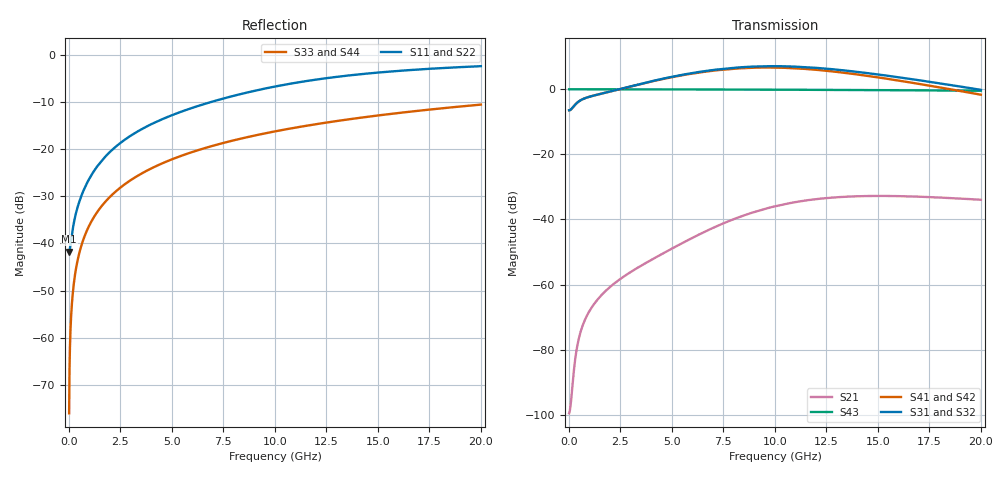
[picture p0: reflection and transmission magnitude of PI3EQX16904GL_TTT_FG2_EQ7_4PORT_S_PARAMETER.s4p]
! NPort=4 DATA=2000 NOISE=0 GROUPDELAY=0 COMPLEX_DATAFORMAT=POLAR
! NumOfBlock=1 NumOfParam=0
! .MODEL Smodel S TSTONEFILE=PI3EQX16904GL_TTT_FG2_EQ7_4PORT_S_PARAMETER.s4p TYPE=S
!  -- The above .MODEL line can be used for the S element in the netlist.
! The s parameter is extracted from the linear redriver, it is not bi-directional; only s(4,1)s(4,2) and s(3,1)s(3,2)
! should be the insertion loss
!Port definition:
!Port1 = input+
!Port2 = input-
!Port3 = output+
!Port4 = output-
# Hz S MA R  50
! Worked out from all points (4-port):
!   2000 points, 10 MHz to 20 GHz, reference 50 ohm
!   strongest paths, dB at 10 MHz, 5.01 GHz, 10.01 GHz, 15.01 GHz, 20 GHz:
!     S31: -6.5, 3.9, 7.1, 4.6, -0.2
!     S32: -6.5, 3.8, 7.1, 4.5, -0.2
!     S41: -6.5, 3.7, 6.7, 3.7, -1.7
!     S42: -6.5, 3.7, 6.6, 3.6, -1.7
!     S43: 0.0, 0.0, -0.1, -0.3, -0.4
!     S21: -99.6, -48.9, -35.9, -32.8, -33.9
!   lowest |S11| = -41.7 dB at 10 MHz (marker M1), VSWR 1.02, Z = 49.2 - j0.0603 ohm
!   |S11| at or under -10 dB: start of sweep to 6.858 GHz
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1e7  0.008182 -175.7  1.05e-05 7.8  0 0.0  0 0.0
     1.05e-05 7.8  0.008182 -175.7  0 0.0  0 0.0
     0.4744 0.7  0.4744 -179.3  0.0001571 -90.0  1 -0.0
     0.4744 -179.3  0.4744 0.7  1 -0.0  0.0001571 -90.0
2.8e8  0.01832 -124.6  6.153e-05 116.3  0 0.0  0 0.0
       6.153e-05 116.3  0.01832 -124.6  0 0.0  0 0.0
       0.5696 14.2  0.5696 -165.8  0.004398 -90.3  1 -0.3
       0.5695 -166.3  0.5696 13.7  1 -0.3  0.004398 -90.3
1.01e9  0.04965 -106.4  0.0003975 112.2  0 0.0  0 0.0
        0.0003974 112.2  0.04965 -106.4  0 0.0  0 0.0
        0.7708 11.7  0.7715 -168.3  0.01586 -90.9  0.9999 -0.9
        0.7704 -170.1  0.771 9.9  0.9999 -0.9  0.01586 -90.9
5.5e9  0.2531 -103.9  0.00436 110.5  0 0.0  0 0.0
       0.004328 110.9  0.2531 -103.9  0 0.0  0 0.0
       1.67 -30.1  1.658 149.5  0.08605 -95.1  0.996 -4.9
       1.644 140.1  1.633 -40.3  0.996 -4.9  0.08605 -95.1
9.41e9  0.4369 -111.2  0.01432 74.7  0 0.0  0 0.0
        0.01423 75.7  0.4368 -111.2  0 0.0  0 0.0
        2.258 -96.8  2.243 83.0  0.1461 -98.7  0.9884 -8.4
        2.162 66.8  2.148 -113.4  0.9884 -8.4  0.1461 -98.7
1.332e10  0.5999 -121.7  0.02231 23.1  0 0.0  0 0.0
          0.02224 24.5  0.6 -121.6  0 0.0  0 0.0
          1.958 -165.7  1.945 14.0  0.2044 -102.3  0.9772 -11.8
          1.801 -8.4  1.789 171.4  0.9772 -11.8  0.2044 -102.3
2e10  0.7643 -136.5  0.02007 -39.0  0 0.0  0 0.0
      0.02008 -37.0  0.7646 -136.5  0 0.0  0 0.0
      0.9812 100.7  0.9731 -79.6  0.2986 -108.1  0.9506 -17.4
      0.8261 -111.2  0.8194 68.4  0.9506 -17.4  0.2986 -108.1
